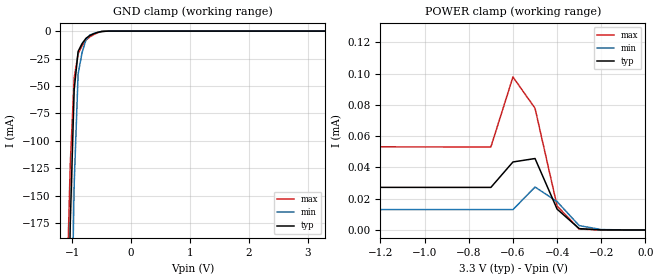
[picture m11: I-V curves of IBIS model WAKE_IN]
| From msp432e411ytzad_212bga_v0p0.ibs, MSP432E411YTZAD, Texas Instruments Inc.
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|   Model Cell WAKE_IN
[Model]   WAKE_IN
Model_type   Input
Polarity   Non-Inverting
Vinl =  0.8
Vinh =  2
C_comp   5.465001p   4.617803p   6.275566p
[Model Spec]
Vinl   0.8   0.8   0.8
Vinh   2   2   2
[Temperature Range]   25   125   -40
[Voltage Range]   3.3   2.97   3.63
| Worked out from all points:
|   GND clamp passes 1 mA (typ) near -0.55 V on its own axis
| Nom Voltages:
|   IBIASFET=3.3, VDDC=1.2, VDD=3.3, GND=0
| Min Voltages:
|   IBIASFET=2.97, VDDC=1.08, VDD=2.97, GND=0
| Max Voltages:
|   IBIASFET=3.63, VDDC=1.32, VDD=3.63, GND=0
[POWER_clamp]
|   voltage   I(typ)   I(min)   I(max)
-3.3V     115.1uA    433.3mA    64.95uA
-3.2V     32.43uA    390.6mA    63.45uA
-3V       29.84uA    305.6mA    60.86uA
-2.033V   27.65uA    244.4uA    54.35uA
-2V       27.61uA    48.33uA    54.25uA
-1.9V     27.53uA    15.07uA    54uA
-700mV    27.24uA    13.03uA    53.12uA
-600mV    43.52uA    13.03uA    97.89uA
-500mV    45.71uA    27.48uA    77.88uA
-400mV    13.32uA    18.12uA    15.3uA
-300mV    859.4nA    2.798uA    598.6nA
0V        395.6pA    9.845nA    58.24pA
[GND_clamp]
|   voltage   I(typ)   I(min)   I(max)
-3.3V     -16.39A    -15.37A    -17.22A
-1.1V     -385.1mA   -635.6mA   -256.3mA
-1.033V   -175.6mA   -338.3mA   -121.2mA
-966.7mV  -53.38mA   -139.4mA   -42.75mA
-900mV    -18.52mA   -39.05mA   -20.75mA
-833.3mV  -11.44mA   -19.73mA   -13.31mA
-766.7mV  -6.599mA   -7.926mA   -8.148mA
-700mV    -3.986mA   -3.644mA   -5.249mA
-500mV    -328.3uA   -388.2uA   -374.5uA
-366.7mV  -15.94uA   -32.84uA   -14.83uA
3.3V      395.6pA    5.294uA    29.38pA
